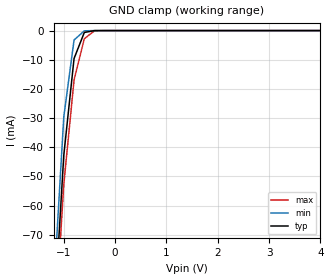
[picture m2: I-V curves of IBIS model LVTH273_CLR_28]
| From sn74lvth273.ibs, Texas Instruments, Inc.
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|   Model LVTH273_CLR_28
[Model]   LVTH273_CLR_28
Model_type  Input
Polarity   Non-Inverting
Vinl = 0.8
Vinh = 2.0
| variable   typ   min   max
C_comp   4pf   NA   NA
[Temperature Range]   40   -25   100
| Ambient temperatur   25   -40   85
[Voltage range]   2.8   2.7   2.9
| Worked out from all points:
|   GND clamp passes 1 mA (typ) near -0.61 V on its own axis
[GND Clamp]
|   Voltage   I(typ)   I(min)   I(max)
-5V       -1.924A    -2.133A    -1.83A
-1.2V     -101.7mA   -89.99mA   -109.9mA
-1V       -42.7mA    -29.54mA   -52.69mA
-800mV    -9.568mA   -3.232mA   -16.91mA
-600mV    -647.2uA   -90.42uA   -2.777mA
-400mV    -2.806uA   -64.26nA   -83.43uA
5V        113.1pA    154.8pA    263pA
